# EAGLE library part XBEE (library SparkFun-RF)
Digi XBee and XBee Pro XBees are tiny blue chips that can communicate wirelessly with each other. They can do simple things, like replacing a couple of wires in serial communication, which is nice when you want to make a remote for your paintball vehicle. SparkFun Products SparkFun XBee Buying Guide SparkFun XBee Explorer USB (WRL-11812) Breakout Board for XBee Module (WRL-8276) SparkFun XBee Explorer Regulated (WRL-11373) SparkFun XBee Explorer Dongle (WRL-11697) SparkFun XBee Shield (WRL-12847) SparkFun XBee Explorer Serial (WRL-13225)
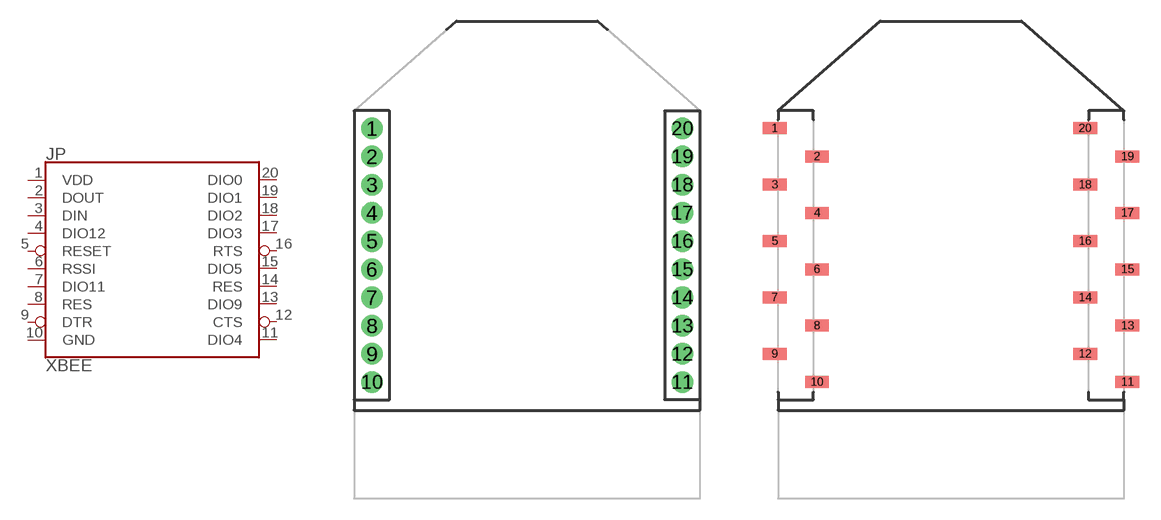
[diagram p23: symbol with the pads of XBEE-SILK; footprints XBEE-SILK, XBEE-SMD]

Designator prefix JP

## XBEESILK  [XBEE-SILK]
1  VDD  pwr
2  DOUT  out
3  DIN  in
4  DIO12
5  RESET  in
6  RSSI
7  DIO11
8  RES
9  DTR
10  GND  pwr
11  DIO4
12  CTS  out
13  DIO9
14  RES
15  DIO5
16  RTS  in
17  DIO3
18  DIO2
19  DIO1
20  DIO0

## XBEESMD (PROD_ID: CONN-09042)  [XBEE-SMD]
Pads as for XBEE-SILK

## XBEELONGPAD  [XBEE-LONGPAD]
Pads as for XBEE-SILK

## XBEELOCK  [XBEE-LOCK]
Pads as for XBEE-SILK

## XBEE  [XBEE]
Pads as for XBEE-SILK

## Footprint XBEE-SILK (pad centres in mm)
Digi XBee and XBee-PRO RF Modules (Silkscreen Dimension Indicators) 20-pin 2mm PTH headers. Silkscreen to indicate polarity and dimensions of XBee (non-Pro's) XBee Mechanical Drawings Header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
drill 0.8 pad 1.524: 1 -11,20; 2 -11,18; 3 -11,16; 4 -11,14; 5 -11,12; 6 -11,10; 7 -11,8; 8 -11,6; 9 -11,4; 10 -11,2; 11 11,2; 12 11,4; 13 11,6; 14 11,8; 15 11,10; 16 11,12; 17 11,14; 18 11,16; 19 11,18; 20 11,20

## Footprint XBEE-SMD (pad centres in mm)
Digi XBee and XBee-PRO RF Modules (SMD pads) 20-pin 2mm SMD headers. XBee Mechanical Drawings Header Mechanical Drawing Header SparkFun Product Link
smd 1.7 x 0.85: 1 -12.5,20; 2 -9.5,18; 3 -12.5,16; 4 -9.5,14; 5 -12.5,12; 6 -9.5,10; 7 -12.5,8; 8 -9.5,6; 9 -12.5,4; 10 -9.5,2; 11 12.5,2; 12 9.5,4; 13 12.5,6; 14 9.5,8; 15 12.5,10; 16 9.5,12; 17 12.5,14; 18 9.5,16; 19 12.5,18; 20 9.5,20

## Footprint XBEE-LONGPAD (pad centres in mm)
Digi XBee and XBee-PRO RF Modules (Long pads) 20-pin 2mm PTH headers. Elongated annular rings to make soldering easier. XBee Mechanical Drawings Header Mechanical Drawing Header SparkFun Product Link
drill 0.8 pad 1.206 long: 1 -11,20; 2 -11,18; 3 -11,16; 4 -11,14; 5 -11,12; 6 -11,10; 7 -11,8; 8 -11,6; 9 -11,4; 10 -11,2; 11 11,2; 12 11,4; 13 11,6; 14 11,8; 15 11,10; 16 11,12; 17 11,14; 18 11,16; 19 11,18; 20 11,20

## Footprint XBEE-LOCK (pad centres in mm)
Digi XBee and XBee-PRO RF Modules (Locking footprint) 20-pin 2mm PTH headers - offset to "lock" headers in place for soldering. XBee Mechanical Drawings Header Mechanical Drawing Header SparkFun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
drill 0.737 pad 1.524: 1 -11.178,20; 2 -10.822,18; 3 -11.178,16; 4 -10.822,14; 5 -11.178,12; 6 -10.822,10; 7 -11.178,8; 8 -10.822,6; 9 -11.178,4; 10 -10.822,2; 11 11.178,2; 12 10.822,4; 13 11.178,6; 14 10.822,8; 15 11.178,10; 16 10.822,12; 17 11.178,14; 18 10.822,16; 19 11.178,18; 20 10.822,20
